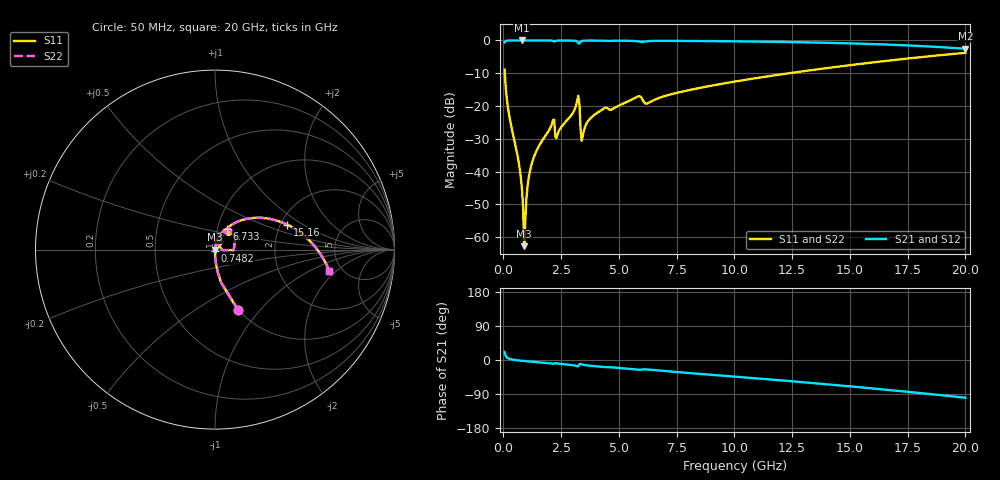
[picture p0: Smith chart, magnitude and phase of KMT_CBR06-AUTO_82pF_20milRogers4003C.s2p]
! Data measured by Modelithics Inc. support@modelithics.com 813-866-6335
! KEMET CBR06-AUTO 82pF, Pad Width= 0.851mm, Pad Length= 0.64mm, Pad Gap= 0.62mm, 20mil Rogers 4003C substrate Data, January 2022
# hz S ma R 50
! 2 Port Network Data from SP1.SP block
! freq  magS11  angS11  magS21  angS21  magS12  angS12  magS22  angS22
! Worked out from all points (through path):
!   401 points, 50 MHz to 20 GHz, reference 50 ohm
!   highest |S21| = 0.00 dB at 798.1 MHz (marker M1); lowest = -2.5 dB at 20 GHz (marker M2)
!   group delay of S21, straight-line fit = 13.8 ps
!   lowest |S11| = -62.7 dB at 897.9 MHz (marker M3), VSWR 1.00, Z = 50 - j0.0567 ohm
!   |S11| at or under -10 dB: 59.91 MHz to 12.36 GHz (12.3 GHz wide, 198 % of centre)
!   |S22| runs from -62.7 to -3.8 dB; largest |S21 - S12| = 0
!   S11 on the Smith chart (normalised r, x): 50 MHz: 1.00, -0.77; 748.2 MHz: 1.00, -0.02; 6.733 GHz: 1.11, +0.26; 15.16 GHz: 2.18, +0.74; 20 GHz: 3.96, -1.64
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5e7  0.3598 -69.0  0.9327 20.9  0.9327 20.9  0.3598 -69.0
2.495e8  0.07156 -86.4  0.9971 3.3  0.9971 3.3  0.07156 -86.4
7.4825e8  0.008431 -88.8  0.9995 -1.8  0.9995 -1.8  0.008431 -88.8
7.98125e8  0.005639 -87.4  0.9995 -2.1  0.9995 -2.1  0.005639 -87.4
8.97875e8  0.0007315 -50.7  0.9995 -2.7  0.9995 -2.7  0.0007315 -50.7
9.97625e8  0.004052 79.4  0.9994 -3.3  0.9994 -3.3  0.004052 79.4
1.097375e9  0.008238 82.4  0.9994 -3.8  0.9994 -3.8  0.008238 82.4
1.296875e9  0.01595 83.0  0.9992 -4.9  0.9992 -4.9  0.01595 83.0
2.094875e9  0.05288 74.9  0.9933 -9.4  0.9933 -9.4  0.05288 74.9
2.34425e9  0.03721 73.3  0.9944 -9.2  0.9944 -9.2  0.03721 73.3
3.192125e9  0.1205 58.1  0.9608 -16.4  0.9608 -16.4  0.1205 58.1
3.391625e9  0.02955 36.7  0.98 -11.6  0.98 -11.6  0.02955 36.7
3.4415e9  0.03611 59.1  0.9878 -12.4  0.9878 -12.4  0.03611 59.1
4.33925e9  0.0913 67.6  0.9894 -18.4  0.9894 -18.4  0.0913 67.6
5.8355e9  0.1407 55.1  0.9675 -25.7  0.9675 -25.7  0.1407 55.1
6.184625e9  0.1085 52.0  0.9694 -24.8  0.9694 -24.8  0.1085 52.0
6.73325e9  0.1327 59.8  0.9858 -28.0  0.9858 -28.0  0.1327 59.8
1.0025e10  0.2365 45.6  0.9688 -43.9  0.9688 -43.9  0.2365 45.6
1.336662e10  0.354 28.7  0.9313 -60.7  0.9313 -60.7  0.354 28.7
1.516212e10  0.4266 18.9  0.8992 -70.4  0.8992 -70.4  0.4266 18.9
1.670825e10  0.4941 10.0  0.8625 -79.3  0.8625 -79.3  0.4941 10.0
2e10  0.6481 -10.7  0.7474 -99.5  0.7474 -99.5  0.6481 -10.7
